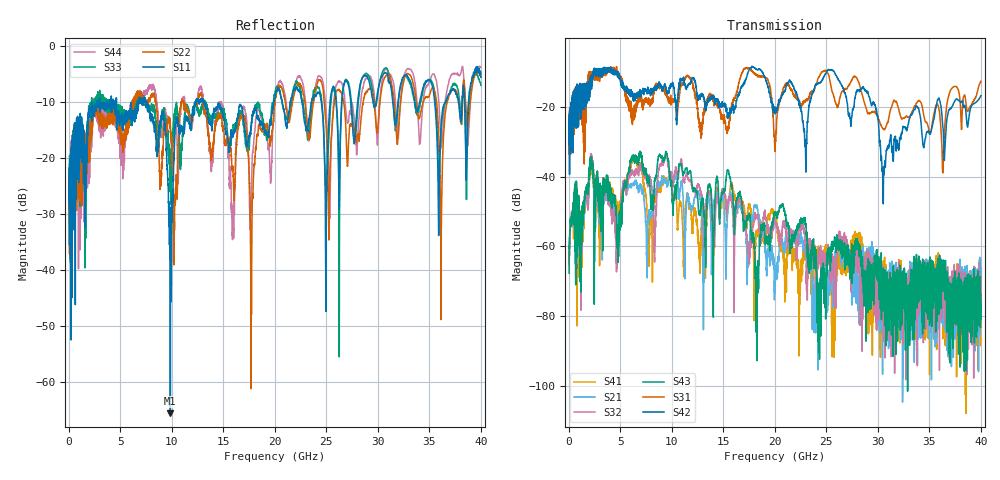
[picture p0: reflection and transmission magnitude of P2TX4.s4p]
!Agilent Technologies,N5245A,MY49151084,A.09.20.08
!Agilent N5245A: A.09.20.08
!Date: Thursday, March 01, 2012 14:19:26
!Correction: S11(Full 4 Port(1,2,3,4))
!S12(Full 4 Port(1,2,3,4))
!S13(Full 4 Port(1,2,3,4))
!S14(Full 4 Port(1,2,3,4))
!S21(Full 4 Port(1,2,3,4))
!S22(Full 4 Port(1,2,3,4))
!S23(Full 4 Port(1,2,3,4))
!S24(Full 4 Port(1,2,3,4))
!S31(Full 4 Port(1,2,3,4))
!S32(Full 4 Port(1,2,3,4))
!S33(Full 4 Port(1,2,3,4))
!S34(Full 4 Port(1,2,3,4))
!S41(Full 4 Port(1,2,3,4))
!S42(Full 4 Port(1,2,3,4))
!S43(Full 4 Port(1,2,3,4))
!S44(Full 4 Port(1,2,3,4))
!S4P File: Measurements: <S11,S12,S13,S14>,
!<S21,S22,S23,S24>,
!<S31,S32,S33,S34>,
!<S41,S42,S43,S44>:
# Hz S  dB  R 50
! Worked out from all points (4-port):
!   3996 points, 50 MHz to 40 GHz, reference 50 ohm
!   strongest paths, dB at 50 MHz, 10.04 GHz, 20.03 GHz, 30.02 GHz, 40 GHz:
!     S42: -26.9, -13.5, -21.4, -23.8, -16.7
!     S31: -25.0, -18.7, -31.8, -22.8, -12.6
!     S43: -67.7, -46.0, -50.9, -65.1, -76.4
!     S32: -63.2, -40.8, -52.7, -67.8, -69.3
!     S21: -59.7, -40.9, -68.7, -72.9, -66.2
!     S41: -59.5, -43.1, -50.8, -82.1, -72.3
!   lowest |S11| = -65.5 dB at 9.87 GHz (marker M1), VSWR 1.00, Z = 50 + j0.0529 ohm
!   |S11| at or under -10 dB: start of sweep to 2.23 GHz; 7.491 GHz to 12.3 GHz (4.809 GHz wide, 48.6 % of centre); 13.12 GHz to 19.9 GHz (6.774 GHz wide, 41 % of centre)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
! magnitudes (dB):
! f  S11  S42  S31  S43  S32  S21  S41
! 50 MHz  -24.8  -26.9  -25.0  -67.7  -63.2  -59.7  -59.5
! 2.18 GHz  -11.6  -14.3  -11.6  -34.3  -33.4  -34.2  -35.4
! 9.87 GHz  -65.5  -13.9  -18.2  -40.9  -40.1  -41.0  -41.4
! 17.73 GHz  -14.4  -8.6  -9.5  -58.0  -58.0  -51.5  -50.9
! 24.02 GHz  -8.8  -13.5  -13.2  -63.4  -71.9  -78.7  -62.1
! 30.56 GHz  -5.0  -37.7  -26.4  -68.4  -75.3  -73.0  -70.7
! 40 GHz  -5.6  -16.7  -12.6  -76.4  -69.3  -66.2  -72.3
